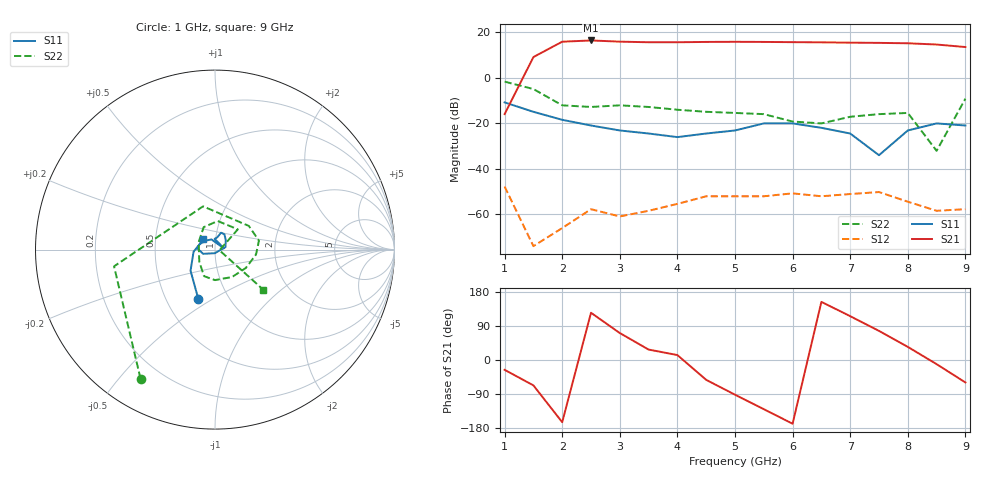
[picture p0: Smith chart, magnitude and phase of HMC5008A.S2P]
! HMMC-5008
! S Parameters  (TA=25C, VDD=5V, IDD=150 mA, Zo=50 Ohms)
# ghz s ma r 50
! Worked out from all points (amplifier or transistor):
!   17 points, 1 GHz to 9 GHz, reference 50 ohm
!   highest |S21| = 16.5 dB at 2.5 GHz (marker M1)
!   |S21| within 3 dB of that: 1.818 GHz to end of sweep
!   unconditionally stable (mu >= 1): start of sweep to end of sweep
!   at 2 GHz: K = 147.59, MAG = 16.3 dB, |S12| = -66.0 dB
!   at 5 GHz: K = 31.02, MAG = 16.0 dB, |S12| = -52.0 dB
!   at 9 GHz: K = 70.04, MAG = 14.2 dB, |S12| = -57.7 dB
1  0.29 -108.7  0.16 -25.9  0.0041 119.3  0.83 -120.0
1.5  0.18 -139.2  2.88 -67.0  0.0002 64.3  0.57 -170.6
2  0.12 -174.4  6.26 -164.1  0.0005 156.5  0.25 105.4
2.5  0.09 159.7  6.67 124.7  0.0013 117.5  0.23 35.0
3  0.07 133.7  6.28 71.1  0.0009 171.6  0.25 11.5
3.5  0.06 109.2  6.09 27.5  0.0012 103.1  0.23 -6.9
4  0.05 8.3  6.09 13.0  0.0017 121.7  0.2 -30.7
4.5  0.06 91.8  6.19 -52.4  0.0025 93.8  0.18 -58.0
5  0.07 79.3  6.23 -91.6  0.0025 89.1  0.17 -90.0
5.5  0.1 70.2  6.19 -129.8  0.0025 79.8  0.16 -112.4
6  0.1 58.3  6.12 -168.1  0.0029 53.6  0.11 -142.7
6.5  0.08 41.5  6.06 153.4  0.0025 54.6  0.1 155.7
7  0.06 13.4  5.97 115.6  0.0028 22.7  0.14 116.7
7.5  0.02 -92.3  5.9 76.8  0.0031 16.3  0.16 84.5
8  0.07 -160.3  5.78 34.6  0.0019 -27.2  0.17 41.6
8.5  0.1 175.8  5.43 -10.9  0.0012 -8.0  0.025 -8.8
9  0.09 137.6  4.78 -59.2  0.0013 71.8  0.35 -39.7
